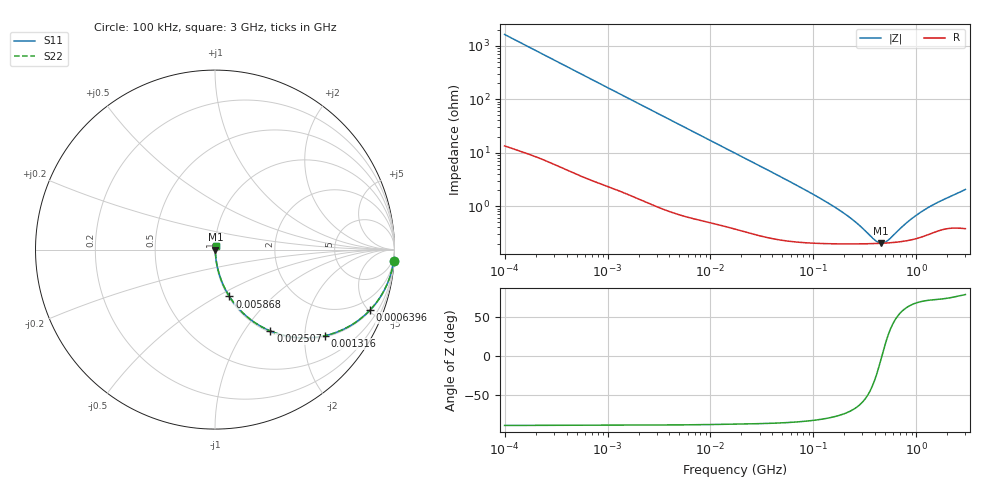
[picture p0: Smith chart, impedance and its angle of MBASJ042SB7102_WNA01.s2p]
! MBASJ042SB7102_WNA01  S-PARAMETER MODEL  ( Standard Model )
! Model Generated by TAIYO YUDEN Corporation (https://www.yuden.co.jp/en/)
! Version 1.0
! TAIYO YUDEN Control No. 250312
! Copyright(c) 2025 TAIYO YUDEN CO.,LTD. All Rights Reserved.
! Product Description (link to TY-COMPAS)
! https://ds.yuden.co.jp/TYCOMPAS/or/detail?pn=MBASJ042SB7102KWNA01&u=M
! Products Name : Multilayer Ceramic Capacitors
! Characteristics :
!  Capacitance : 1000 [pF] , Rated Voltage : 6.3 [V] , TCC : X7R
!  Case Size : 0.4 x 0.2 / 0.016 x 0.008 [mm/inch] , Thickness : 0.2 / 0.008 [mm/inch]
!  (Conditions: Temperature = 25 [degC] , DC Bias Voltage = 0 [V])
! External Node Assignments :
!  1  o---| |---o  2
! GND o---------o GND
! Frequency Range : 100kHz  -  3GHz  [ 401 STEP ]
# MHZ S RI R 50
! Freq[MHz].  S11 Real  S11 Imag  S21 Real  S21 Imag  S12 Real  S12 Imag  S22 Real  S22 Imag
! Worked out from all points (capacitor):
!   401 points, 100 kHz to 3 GHz, reference 50 ohm
!   read as one part in series: C = 980 pF near 105.3 kHz
!   lowest |Z| = 202 mohm at 457.1 MHz (marker M1)
!   series resonance near 463 MHz, so ESL is about 120 pH
!   S11 on the Smith chart (normalised r, x): 100 kHz: 1, -32; 639.6 kHz: 1.06, -5.14; 1.316 MHz: 1.04, -2.51; 2.507 MHz: 1.02, -1.33; 5.868 MHz: 1.01, -0.57; 3 GHz: 1.01, +0.04
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0.1  0.9957 -0.0613  0.00429 0.0613  0.00429 0.0613  0.9957 -0.0613
0.246461  0.9762 -0.1472  0.0238 0.1472  0.0238 0.1472  0.9762 -0.1472
0.562235  0.892 -0.3043  0.108 0.3043  0.108 0.3043  0.892 -0.3043
0.639561  0.8653 -0.3352  0.1347 0.3352  0.1347 0.3352  0.8653 -0.3352
0.917447  0.7602 -0.4201  0.2398 0.4201  0.2398 0.4201  0.7602 -0.4201
1.316074  0.6103 -0.4802  0.3897 0.4802  0.3897 0.4802  0.6103 -0.4802
1.793056  0.4614 -0.4905  0.5386 0.4905  0.5386 0.4905  0.4614 -0.4905
2.506689  0.3086 -0.4535  0.6914 0.4535  0.6914 0.4535  0.3086 -0.4535
3.161081  0.2215 -0.4064  0.7785 0.4064  0.7785 0.4064  0.2215 -0.4064
5.867632  0.0802 -0.2608  0.9198 0.2608  0.9198 0.2608  0.0802 -0.2608
10.08119  0.0316 -0.1609  0.9684 0.1609  0.9684 0.1609  0.0316 -0.1609
17.7727  0.0126 -0.0939  0.9874 0.0939  0.9874 0.0939  0.0126 -0.0939
97.38194  0.00232 -0.0169  0.9977 0.0169  0.9977 0.0169  0.00232 -0.0169
205.6221  0.00201 -0.00671  0.998 0.00671  0.998 0.00671  0.00201 -0.00671
273.0175  0.00198 -0.00411  0.998 0.00411  0.998 0.00411  0.00198 -0.00411
391.6425  0.002 -0.00125  0.998 0.00125  0.998 0.00125  0.002 -0.00125
457.1373  0.00202 -9.46e-05  0.998 9.46e-05  0.998 9.46e-05  0.00202 -9.46e-05
547.5153  0.00206 0.00125  0.9979 -0.00125  0.9979 -0.00125  0.00206 0.00125
805.9132  0.00227 0.00433  0.9977 -0.00433  0.9977 -0.00433  0.00227 0.00433
1156.079  0.00274 0.00767  0.9973 -0.00767  0.9973 -0.00767  0.00274 0.00767
1616.196  0.00353 0.0112  0.9965 -0.0112  0.9965 -0.0112  0.00353 0.0112
3000  0.00419 0.02  0.9958 -0.02  0.9958 -0.02  0.00419 0.02
